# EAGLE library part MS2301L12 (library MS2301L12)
SLIDE SWITCH DP3T 200MA 30VDC Source: Datasheet
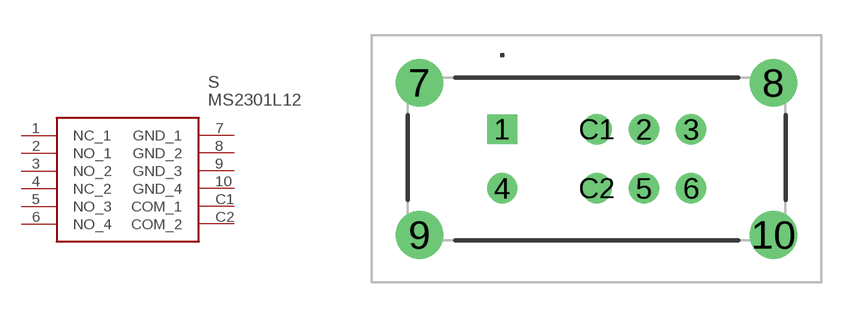
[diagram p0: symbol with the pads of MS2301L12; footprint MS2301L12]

Designator prefix S

## MS2301L12 (Description: SLIDE SWITCH DP3T 200MA 30VDC; Height: 20.1mm; Manufacturer_Name: CIT Relay & Switch; Manufacturer_Part_Number: MS2301L12)  [MS2301L12]
1  NC_1
2  NO_1
3  NO_2
4  NC_2
5  NO_3
6  NO_4
7  GND_1
8  GND_2
9  GND_3
10  GND_4
C1  COM_1
C2  COM_2

## Footprint MS2301L12 (pad centres in mm)
MS2301L12
drill 0.75 pad 1.2 square: 1 0,0
drill 0.75 pad 1.286: 2 6,0; 3 8,0; 4 0,-2.5; 5 6,-2.5; 6 8,-2.5; C1 4,0; C2 4,-2.5
drill 1.35 pad 2.025: 7 -3.51,1.975; 8 11.49,1.975; 9 -3.51,-4.475; 10 11.49,-4.475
